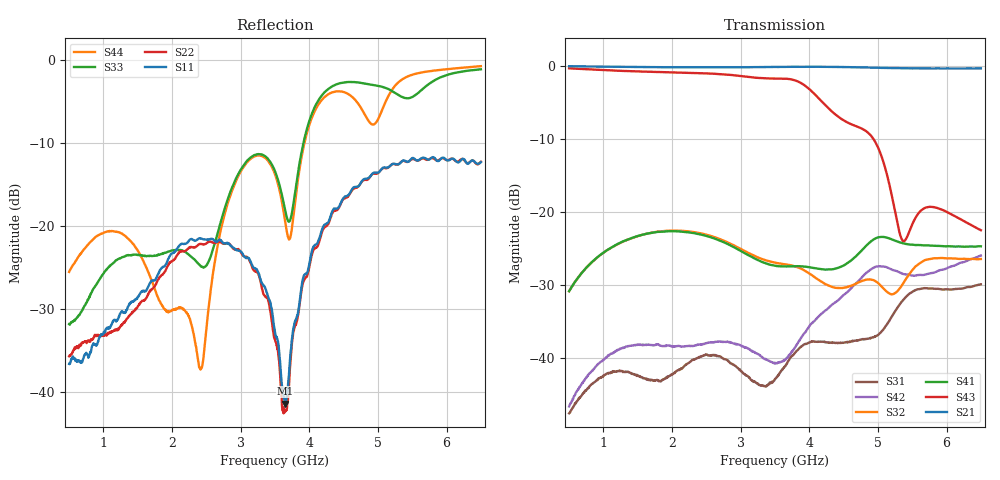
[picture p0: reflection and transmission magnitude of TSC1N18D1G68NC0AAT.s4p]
! TSC1N18D1G68NC0AAT  S-PARAMETER MODEL  ( General Type )
! Model Generated by TAIYO YUDEN Corporation (https://www.yuden.co.jp/en/)
! Version 1.0
! TAIYO YUDEN Control No. 20140626
! Copyright(c) 2014 TAIYO YUDEN CO.,LTD. All Rights Reserved.
! Products Name : Multilayer Ceramic Devices
! Characteristics :
!  Passband freq : 698-2690MHz ( At Passband , Insertion Loss : 0.3dB , VSWR 1.67 ),
!  Coupling : 21.5dB min 29dB max at 698-2690MHz , Directivity : - ,
!  Case Size : 1.6 x 0.8 / 0.063 x 0.031 [mm/inch] , Thickness : 0.65 / 0.026 [mm/inch]
!  (Conditions: Temperature = 25 degC , DC Bias Current/Voltage = 0A / 0V)
! External Node Assignments :
! PIN No.1 Coupling(PORT4)  o---|-------|---o  PIN No.6 Input(PORT1)
! PIN No.2 GND  o---|  |---o  PIN No.5 GND
! PIN No.3 Isolation(PORT3)  o---|-------|---o  PIN No.4 Output(PORT2)
! Frequency Range : 500MHz  -  6.5GHz  [ 6001 STEP ]
# MHz S RI R 50
! Freq[MHz].  S11 Real  S11 Imag  S12 Real  S12 Imag  S13 Real  S13 Imag  S14 Real  S14 Imag
!  S21 Real  S21 Imag  S22 Real  S22 Imag  S23 Real  S23 Imag  S24 Real  S24 Imag
!  S31 Real  S31 Imag  S32 Real  S32 Imag  S33 Real  S33 Imag  S34 Real  S34 Imag
!  S41 Real  S41 Imag  S42 Real  S42 Imag  S43 Real  S43 Imag  S44 Real  S44 Imag
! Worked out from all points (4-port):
!   6001 points, 500 MHz to 6.5 GHz, reference 50 ohm
!   strongest paths, dB at 500 MHz, 2 GHz, 3.5 GHz, 5 GHz, 6.5 GHz:
!     S21: -0.1, -0.2, -0.2, -0.3, -0.4
!     S43: -0.4, -0.9, -1.7, -11.2, -22.5
!     S41: -30.8, -22.6, -27.3, -23.5, -24.7
!     S32: -30.8, -22.6, -26.9, -29.7, -26.4
!     S42: -46.6, -38.4, -40.7, -27.4, -26.0
!     S31: -47.5, -42.2, -42.8, -36.8, -29.9
!   lowest |S11| = -41.3 dB at 3.645 GHz (marker M1), VSWR 1.02, Z = 50.7 - j0.453 ohm
!   |S11| at or under -10 dB: start of sweep to end of sweep
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500  0.00725 0.0129  0.988 -0.1119  0.00183 0.00374  0.0123 0.0259
     0.9869 -0.1115  0.0107 0.0126  0.0117 0.0262  0.00177 0.00437
     0.00184 0.00377  0.0117 0.0262  0.00533 -0.0252  0.716 -0.6383
     0.0123 0.0259  0.00172 0.00435  0.7168 -0.6388  0.0257 -0.0466
2039  0.00525 -0.0699  0.892 -0.3972  0.00777 -0.00176  0.0707 -0.0213
      0.8918 -0.3971  -0.000257 -0.0636  0.0741 -0.00743  0.00856 -0.0085
      0.00772 -0.00177  0.0742 -0.00745  0.0689 -0.0203  -0.9003 0.000629
      0.0706 -0.0213  0.00854 -0.00845  -0.8994 0.000381  -0.0154 -0.0276
2859  -0.0148 -0.0748  0.8198 -0.5317  -0.00109 -0.00909  0.0171 -0.0562
      0.8185 -0.5313  -0.0268 -0.0716  0.0409 -0.0443  -0.00488 -0.0118
      -0.00106 -0.00915  0.0409 -0.0444  0.1638 -0.0205  0.00672 0.865
      0.0173 -0.0562  -0.0049 -0.0118  0.0066 0.8652  0.1565 -0.0188
3645  0.00731 -0.00447  0.73 -0.6588  0.00377 0.00795  -0.0326 -0.027
      0.7294 -0.6573  0.00682 -0.00332  0.000687 -0.0439  -0.000891 0.00966
      0.00376 0.00796  0.0006 -0.0439  0.085 -0.0938  0.7994 -0.168
      -0.0325 -0.0271  -0.00092 0.00971  0.7989 -0.1682  0.0522 -0.0958
4872  0.1472 0.131  0.5298 -0.8133  -0.00948 -0.00984  -0.0443 0.0424
      0.5294 -0.815  0.1597 0.1123  -0.0266 0.0223  -0.0382 0.011
      -0.00953 -0.00977  -0.0264 0.0223  0.1132 -0.7085  -0.2903 0.1815
      -0.0444 0.0424  -0.0381 0.0109  -0.2916 0.1808  -0.4268 -0.0161
5348  0.1998 0.1442  0.4483 -0.8505  -0.0227 0.00894  -0.0142 0.0598
      0.4478 -0.8511  0.2118 0.1259  -0.0208 0.0236  0.0333 0.0185
      -0.0226 0.00908  -0.0207 0.0236  -0.6029 -0.00637  -0.00646 0.0647
      -0.0142 0.0597  0.0332 0.0184  -0.00665 0.0646  0.764 0.0517
6500  0.2278 0.0865  0.2556 -0.9253  0.0289 -0.0134  0.00101 0.0579
      0.2548 -0.9247  0.229 0.087  0.000629 0.0475  0.00374 -0.0501
      0.0291 -0.0134  0.000413 0.0476  0.7531 -0.4628  0.0633 0.0404
      0.000922 0.0582  0.00374 -0.0503  0.0635 0.04  0.0589 -0.9211
